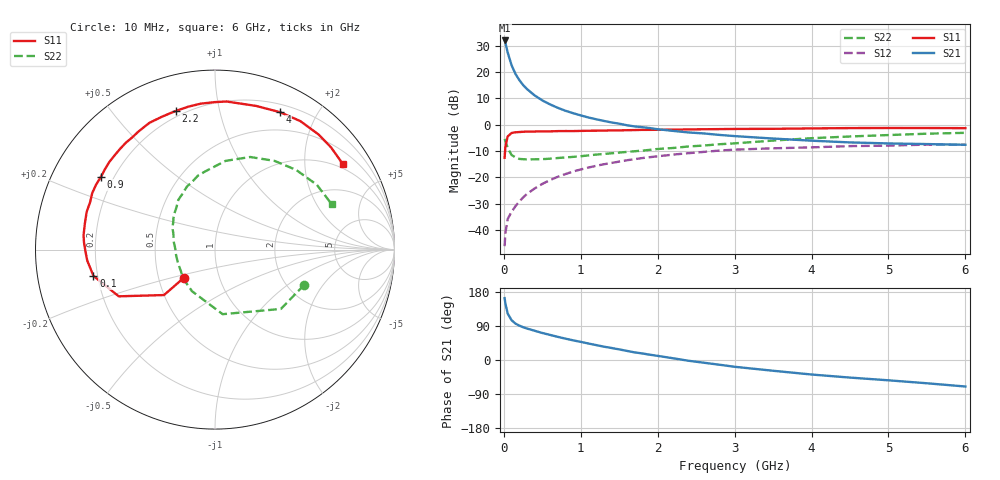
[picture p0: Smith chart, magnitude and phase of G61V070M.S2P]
! SIEMENS Small Signal Semiconductors
! BFG193
! Si NPN RF Bipolar Junction Transistor in SOT223
! VCE = 1 V  IC = 70 mA
! Common Emitter S-Parameters:  August  1996
# GHz  S  MA  R  50
!  f  S11  S21  S12  S22
! GHz  MAG  ANG  MAG  ANG  MAG  ANG  MAG  ANG
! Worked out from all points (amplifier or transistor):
!   36 points, 10 MHz to 6 GHz, reference 50 ohm
!   highest |S21| = 32.0 dB at 10 MHz (marker M1)
!   |S21| within 3 dB of that: start of sweep to 37.02 MHz
!   unconditionally stable (mu >= 1): start of sweep to 23.18 MHz; 116.8 MHz to end of sweep
!   at 250 MHz: K = 1.17, MAG = 18.9 dB, |S12| = -27.7 dB
!   at 1.4 GHz: K = 1.21, MAG = 5.0 dB, |S12| = -14.6 dB
!   at 6 GHz: K = 1.08, MAG = -1.7 dB, |S12| = -7.7 dB
!   S11 on the Smith chart (normalised r, x): 10 MHz: 0.67, -0.22; 100 MHz: 0.18, -0.10; 900 MHz: 0.15, +0.29; 2.2 GHz: 0.17, +0.74; 4 GHz: 0.28, +1.54; 6 GHz: 0.85, +3.06
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0.01  0.2346 -137.8  39.76 163.3  0.0049 68.0  0.5343 -21.6
0.02  0.3807 -138.3  35.81 149.3  0.0087 63.5  0.4941 -42.0
0.05  0.596 -154.1  23.43 122.6  0.0161 54.9  0.3624 -83.2
0.1  0.693 -167.8  13.53 105.1  0.0219 56.5  0.2648 -119.0
0.15  0.7145 -175.1  9.259 96.2  0.0281 58.9  0.2397 -138.2
0.2  0.7228 -179.7  7.065 90.8  0.0344 61.7  0.2233 -149.0
0.25  0.7311 176.8  5.665 86.6  0.0412 63.7  0.2203 -158.3
0.3  0.7368 173.6  4.757 83.1  0.0481 65.0  0.2184 -163.4
0.4  0.7394 168.7  3.594 77.2  0.0611 65.2  0.2193 -173.1
0.5  0.7453 163.6  2.886 71.3  0.0747 64.0  0.2208 -180.0
0.6  0.7442 159.3  2.424 66.2  0.0884 62.9  0.2251 175.0
0.7  0.7531 155.3  2.09 61.1  0.1019 61.4  0.2319 170.6
0.9  0.7537 147.4  1.65 51.9  0.1285 57.2  0.2438 161.5
1.1  0.765 140.3  1.366 43.5  0.1528 52.7  0.2603 154.8
1.6  0.783 123.4  0.974 24.0  0.2103 40.1  0.303 138.3
2.2  0.8024 105.9  0.76 4.6  0.2694 24.6  0.3597 120.3
2.8  0.8218 90.1  0.638 -12.4  0.3211 9.4  0.4237 102.8
3.5  0.8327 74.0  0.544 -28.4  0.3549 -8.9  0.4979 83.2
4  0.8469 64.7  0.495 -38.3  0.3696 -18.6  0.552 69.2
4.5  0.8594 56.4  0.459 -46.4  0.3907 -28.4  0.5954 56.1
5.5  0.8616 41.4  0.427 -61.4  0.4172 -50.5  0.6724 32.5
6  0.8571 34.0  0.414 -70.0  0.4132 -63.0  0.6983 21.1
